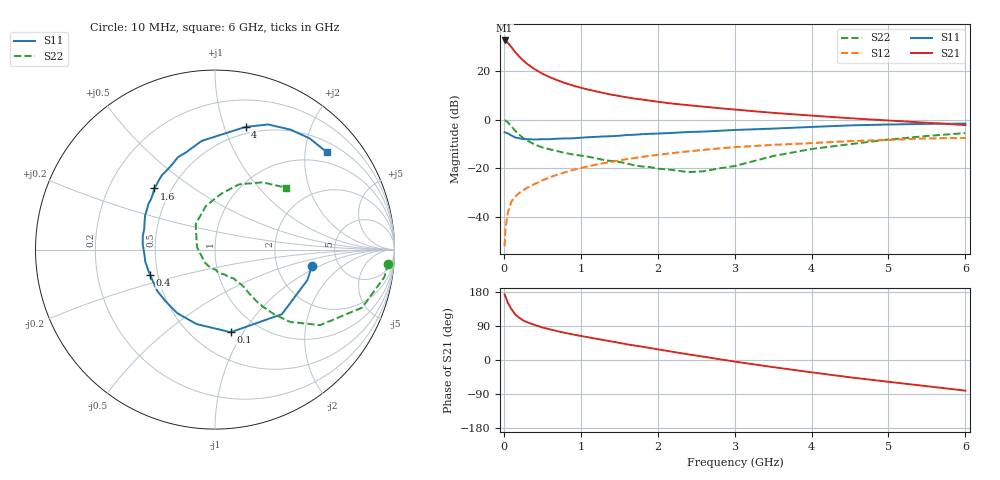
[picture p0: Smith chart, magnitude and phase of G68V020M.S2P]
! SIEMENS Small Signal Semiconductors
! BFG193
! Si NPN RF Bipolar Junction Transistor in SOT223
! VCE = 8 V  IC = 20 mA
! Common Emitter S-Parameters:  August  1996
# GHz  S  MA  R  50
!  f  S11  S21  S12  S22
! GHz  MAG  ANG  MAG  ANG  MAG  ANG  MAG  ANG
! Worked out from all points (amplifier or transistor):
!   36 points, 10 MHz to 6 GHz, reference 50 ohm
!   highest |S21| = 32.5 dB at 10 MHz (marker M1)
!   |S21| within 3 dB of that: start of sweep to 104.8 MHz
!   unconditionally stable (mu >= 1): 742.4 MHz to 2.525 GHz
!   at 250 MHz: K = 0.73, MSG = 26.7 dB, |S12| = -29.1 dB
!   at 1.4 GHz: K = 1.05, MAG = 12.4 dB, |S12| = -17.4 dB
!   at 6 GHz: K = 0.87, MSG = 2.7 dB, |S12| = -7.6 dB
!   S11 on the Smith chart (normalised r, x): 10 MHz: 3.20, -0.81; 100 MHz: 0.75, -0.88; 400 MHz: 0.45, -0.15; 1.6 GHz: 0.40, +0.36; 4 GHz: 0.44, +1.18; 6 GHz: 0.73, +2.48
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0.01  0.5485 -9.3  42.13 173.3  0.0025 90.2  0.9672 -4.6
0.02  0.5421 -18.3  41.57 168.4  0.0053 80.5  0.956 -9.2
0.05  0.518 -44.0  37.96 151.9  0.012 72.9  0.8815 -21.5
0.1  0.4686 -79.2  30.51 133.7  0.0208 64.3  0.7212 -35.7
0.15  0.4275 -103.9  24.05 119.8  0.0264 59.4  0.5812 -43.9
0.2  0.412 -120.8  19.68 111.5  0.0308 58.9  0.4901 -47.5
0.25  0.3984 -133.9  16.39 104.8  0.0352 58.1  0.418 -49.9
0.3  0.3955 -144.4  14.03 99.8  0.0394 59.2  0.373 -51.2
0.4  0.3887 -158.4  10.84 92.5  0.0474 60.5  0.3065 -52.1
0.5  0.3941 -169.9  8.754 85.9  0.0562 60.5  0.2677 -52.2
0.6  0.395 -177.4  7.391 80.8  0.065 60.8  0.2433 -53.0
0.7  0.4041 175.6  6.383 75.9  0.0741 60.2  0.2236 -54.6
0.9  0.411 163.7  4.99 67.3  0.0921 58.0  0.1913 -57.0
1.1  0.4339 153.8  4.111 59.8  0.1094 55.5  0.1713 -63.7
1.6  0.4806 134.8  2.855 41.5  0.1536 46.7  0.1249 -83.4
2.2  0.5318 116.5  2.118 21.4  0.2052 34.6  0.0917 -126.4
2.8  0.5872 101.3  1.713 2.2  0.2551 21.6  0.0993 173.9
3.5  0.6508 84.8  1.371 -18.8  0.3016 5.0  0.1778 127.3
4  0.7043 76.0  1.205 -32.5  0.3275 -4.6  0.2476 102.0
4.5  0.7575 67.0  1.064 -45.7  0.3602 -14.8  0.312 83.9
5.5  0.8138 49.6  0.859 -69.1  0.4098 -38.2  0.4591 54.7
6  0.8261 41.1  0.77 -80.9  0.4171 -51.8  0.5259 41.0
